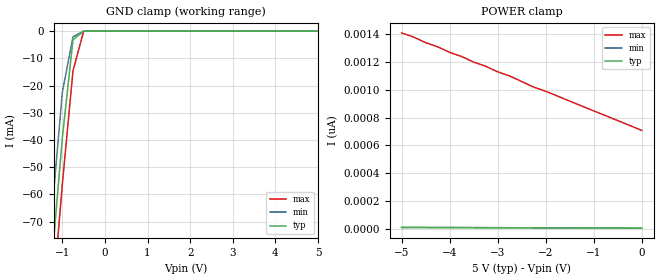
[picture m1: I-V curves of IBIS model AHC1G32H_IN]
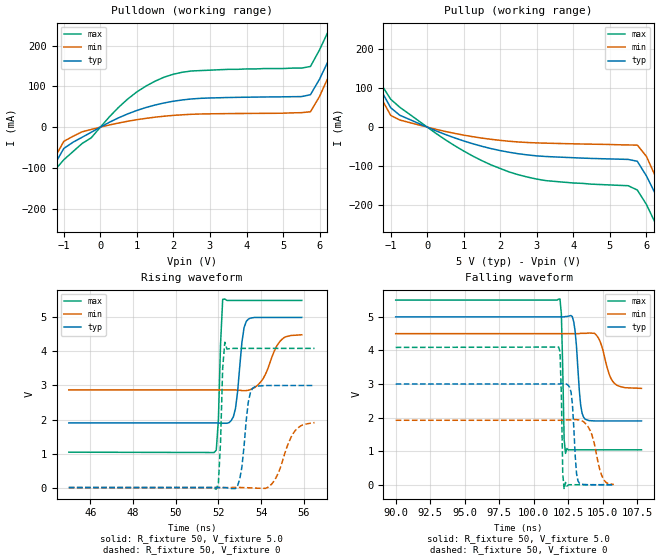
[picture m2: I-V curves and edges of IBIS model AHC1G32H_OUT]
| TEXAS INSTRUMENTS INCORPORATED
| Standard Linear and Logic Group
| IBIS Model of SN74AHC1G32H
| SINGLE 2-INPUT POSITIVE-NOR GATE
| CMPAK-5 5-pin (DCK) Package
[IBIS Ver]   2.1
[Comment Char]  |_char
[File name]   ul32_5c.ibs
[File Rev]   2.0
[Date]   April 17, 2000
[Source]   Data created from SPICE simulations at Hitachi,Ltd.
[Notes]   The following is an IBIS List for the AHC1G32H.
|   Please contact sllibis@ti.com with questions and
|   comments concerning SLL IBIS models.
[Disclaimer] Property of Texas Instruments Incorporated.  Unauthorized
   reproduction and/or distribution is strictly prohibited.
   This product is protected under copyright law.
   Created 2000, (C) Copyright 2000, Texas Instruments Inc.,
   All Rights Reserved.
   UNLESS THERE IS A SIGNED, WRITTEN AGREEMENT TO THE
   CONTRARY, TEXAS INSTRUMENTS () IS PROVIDING THE IBIS
   MODELS  AND WITHOUT ANY WARRANTY, EXPRESSED OR
   IMPLIED.  TI assumes no liability for:
   1) the accuracy of the IBIS models provided to your
   company;
   2) the proper functioning of these IBIS Models in your
   design or for any resulting applications; or
   3) infringement of patents, copyrights or intellectual
   property rights resulting from your use of these IBIS
   models.
   TI provides IBIS Models as a service to our customers.
   You and your company shall not distribute, sell or give
   these models to anyone else without prior written
   permission from TI.
   TI reserves the right to make changes to our products or
   to discontinue any semiconductor product or service
   without notice, and advises our customers to obtain the
   latest version of relevant information to verify, before
   placing orders, that the information being relied on is
   current.
   Please be aware that your receipt and use of the IBIS
   information provided shall serve as acceptance of these
   terms and conditions.  If you do not accept these terms,
   you should return or destroy the IBIS models and any
   other accompanying information immediately.
|   Component AHC1G32H
[Component]   AHC1G32H
[Manufacturer]   Hitachi, Ltd.
[Package]
|   typ   min   max
R_pkg   0.090   0.051   0.105
L_pkg   1.500nH   0.940nH   1.700nH
C_pkg   0.170pF   0.110pF   0.360pF
[Pin]   signal_name   model_name   R_pin   L_pin   C_pin
1   A   AHC1G32H_IN   0.098   1.590nH   0.110pF
2   B   AHC1G32H_IN   0.051   0.940nH   0.170pF
3   GND   GND   0.092   1.590nH   0.360pF
4   Y   AHC1G32H_OUT   0.105   1.700nH   0.110pF
5   VCC   POWER   0.104   1.690nH   0.110pF
| Models and submodels in the file (2): AHC1G32H_IN (Input), AHC1G32H_OUT (Output)
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|   Model AHC1G32H_IN
[Model]   AHC1G32H_IN
Model_type  Input
Polarity   Inverting
Vinl = 1.50
Vinh = 3.50
| variable   typ   min   max
C_comp   2.19pF   2.07pF   2.30pF
[Temperature Range]   25   85   -40
[Voltage Range]   5.0   4.5   5.5
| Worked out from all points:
|   GND clamp passes 1 mA (typ) near -0.58 V on its own axis
[GND Clamp]
|   Voltage   I(typ)   I(min)   I(max)
-5V       -823mA     -807mA     -840mA
-1.5V     -133mA     -115mA     -150mA
-1.25V    -85.2mA    -67.5mA    -103mA
-1V       -39.2mA    -22.5mA    -56.2mA
-750mV    -3.18mA    -2.09mA    -14.6mA
-500mV    -11.6uA    -2.99uA    -57.1uA
5V        5.34pA     5pA        708pA
[POWER Clamp]
|   Voltage   I(typ)   I(min)   I(max)
-5V       10.6pA     10pA       1.41nA
-4.75V    10.3pA     9.75pA     1.38nA
-4.5V     10pA       9.5pA      1.34nA
-4.25V    9.78pA     9.25pA     1.31nA
-4V       9.52pA     9pA        1.27nA
-3.75V    9.26pA     8.75pA     1.24nA
-3.5V     9pA        8.5pA      1.2nA
-3.25V    8.74pA     8.25pA     1.17nA
-2.75V    8.21pA     7.75pA     1.1nA
-2.25V    7.69pA     7.25pA     1.02nA
-2V       7.43pA     7pA        990pA
0V        5.34pA     5pA        708pA
|   Model AHC1G32H_OUT
[Model]   AHC1G32H_OUT
Model_type  Output
Polarity   Inverting
Vmeas = 2.5
Cref = 15pf
| variable   typ   min   max
C_comp   4.52pF   4.32pF   4.72pF
[Temperature Range]   25   85   -40
[Voltage Range]   5.0   4.5   5.5
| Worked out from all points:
|   slope of the pulldown table from 0 to 0.75 V, typ, clamps not added: 23 ohm
|   slope of the pullup table from 0 to 0.75 V, typ, clamps not added: 27.3 ohm
|   rising waveform, R_fixture 50, V_fixture 5.0: 20-80 % time 288ps typ, 654ps min, 137ps max; typ from 1.9 V to 5 V
|   falling waveform, R_fixture 50, V_fixture 5.0: 20-80 % time 325ps typ, 673ps min, 143ps max; typ from 5 V to 1.9 V
|   falling waveform, R_fixture 50, V_fixture 0: 20-80 % time 249ps typ, 665ps min, 126ps max; typ from 3 V to 0 V
|   rising waveform, R_fixture 50, V_fixture 0: 20-80 % time 282ps typ, 677ps min, 132ps max; typ from 0 V to 3 V
[Pulldown]
|   Voltage   I(typ)   I(min)   I(max)
-5V       -826mA     -810mA     -842mA
-2.25V    -282mA     -267mA     -299mA
-2V       -234mA     -219mA     -250mA
-1.25V    -91.3mA    -75.2mA    -106mA
-1V       -52.3mA    -34.7mA    -80mA
750mV     32.6mA     14.5mA     69.2mA
1.75V     59.5mA     26.9mA     123mA
5.75V     79.6mA     37.8mA     149mA
6.25V     165mA      125mA      238mA
6.75V     261mA      217mA      336mA
7V        310mA      265mA      385mA
10V       906mA      861mA      980mA
[Pullup]
|   Voltage   I(typ)   I(min)   I(max)
-5V       828mA      811mA      845mA
-2.25V    284mA      267mA      301mA
-2V       235mA      218mA      252mA
-1V       49.6mA     30.1mA     71.4mA
750mV     -27.5mA    -16mA      -47.4mA
2.25V     -64.5mA    -36.2mA    -115mA
5.75V     -87.4mA    -46mA      -161mA
6V        -125mA     -75mA      -198mA
6.25V     -172mA     -127mA     -247mA
6.75V     -269mA     -224mA     -345mA
7V        -318mA     -273mA     -395mA
10V       -917mA     -874mA     -991mA
[Ramp]
| variable   typ   min   max
dV/dt_r   1.80E+00/2.80E-10   1.15E+00/6.80E-10   2.45E+00/1.30E-10
dV/dt_f   1.86E+00/3.20E-10   9.76E-01/6.70E-10   2.68E+00/1.40E-10
R_load = 50
[Rising Waveform]
R_fixture = 50
V_fixture = 5.0
V_fixture_min = 4.5
V_fixture_max = 5.5
|   Time   V(typ)   V(min)   V(max)
45ns      1.9V       2.87V      1.04V
51.8ns    1.9V       2.87V      1.03V
51.9ns    1.9V       2.87V      1.1V
52ns      1.9V       2.87V      2V
52.1ns    1.89V      2.87V      4.22V
52.2ns    1.89V      2.87V      5.53V
52.8ns    2.33V      2.87V      5.5V
53.3ns    4.88V      2.85V      5.5V
54.9ns    5V         4.31V      5.5V
55.9ns    5V         4.49V      5.5V
[Falling Waveform]
R_fixture = 50
V_fixture = 5.0
V_fixture_min = 4.5
V_fixture_max = 5.5
|   Time   V(typ)   V(min)   V(max)
90ns      5V         4.5V       5.5V
101.9ns   5V         4.5V       5.53V
102ns     5V         4.5V       5.08V
102.2ns   5V         4.5V       1.34V
102.3ns   5.01V      4.5V       934mV
102.9ns   4.84V      4.5V       1.04V
103.4ns   2.36V      4.51V      1.04V
103.7ns   1.96V      4.51V      1.04V
105.8ns   1.9V       3.04V      1.04V
107.8ns   1.9V       2.87V      1.04V
[Falling Waveform]
R_fixture = 50
V_fixture = 0
|   Time   V(typ)   V(min)   V(max)
90ns      3V         1.92V      4.09V
101.8ns   3V         1.92V      4.1V
101.9ns   3V         1.92V      3.96V
102ns     3.01V      1.92V      2.66V
102.1ns   3.01V      1.92V      319mV
102.2ns   3.01V      1.92V      -132mV
102.7ns   2.76V      1.93V      -156uV
103.2ns   117mV      1.93V      124uV
105ns     -303uV     203mV      99uV
105.8ns   -190uV     9.35mV     79uV
[Rising Waveform]
R_fixture = 50
V_fixture = 0
|   Time   V(typ)   V(min)   V(max)
45ns      0V         0V         0V
51.9ns    292uV      -18uV      -47.3mV
52ns      863uV      -20uV      133mV
52.1ns    1.34mV     -23uV      1.34V
52.2ns    1.12mV     -31uV      3.52V
52.3ns    -2.23mV    -9uV       4.27V
53ns      253mV      1.17mV     4.09V
53.4ns    2.52V      -5.51mV    4.09V
53.6ns    2.92V      -11.4mV    4.09V
56.5ns    3V         1.91V      4.09V
